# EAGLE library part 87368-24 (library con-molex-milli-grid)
RECEPTACAL
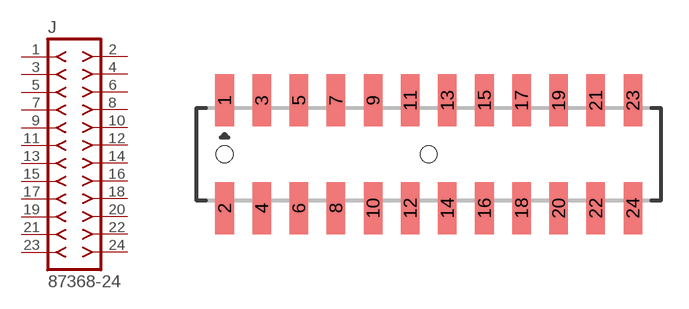
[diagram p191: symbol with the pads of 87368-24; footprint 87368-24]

Designator prefix J

## 87368-24  [87368-24]
1  1  pas
2  2  pas
3  3  pas
4  4  pas
5  5  pas
6  6  pas
7  7  pas
8  8  pas
9  9  pas
10  10  pas
11  11  pas
12  12  pas
13  13  pas
14  14  pas
15  15  pas
16  16  pas
17  17  pas
18  18  pas
19  19  pas
20  20  pas
21  21  pas
22  22  pas
23  23  pas
24  24  pas

## Footprint 87368-24 (pad centres in mm)
RECEPTACAL SMD Dual Row, Side Entry
smd 1 x 2.8: 1 -11,2.9; 2 -11,-2.9; 3 -9,2.9; 4 -9,-2.9; 5 -7,2.9; 6 -7,-2.9; 7 -5,2.9; 8 -5,-2.9; 9 -3,2.9; 10 -3,-2.9; 11 -1,2.9; 12 -1,-2.9; 13 1,2.9; 14 1,-2.9; 15 3,2.9; 16 3,-2.9; 17 5,2.9; 18 5,-2.9; 19 7,2.9; 20 7,-2.9; 21 9,2.9; 22 9,-2.9; 23 11,2.9; 24 11,-2.9
hole 0.914 at -11,0
hole 0.914 at 0,0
